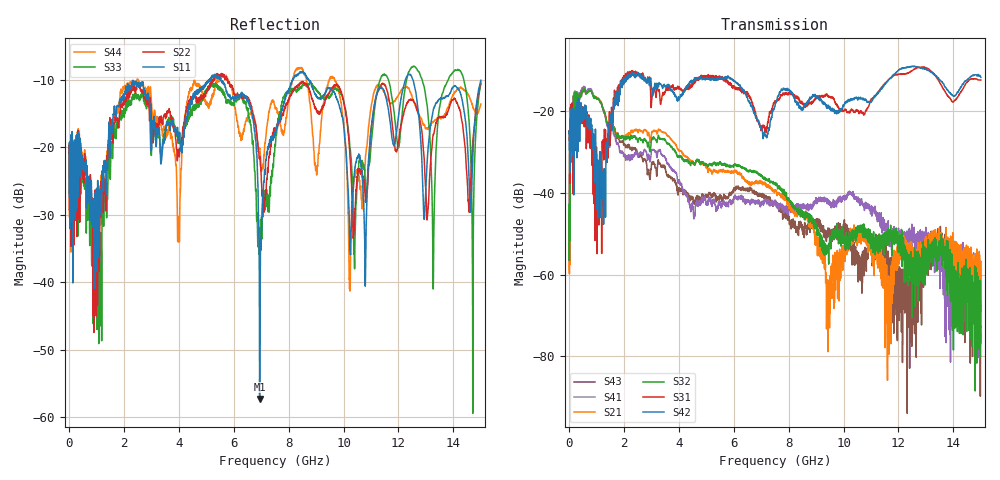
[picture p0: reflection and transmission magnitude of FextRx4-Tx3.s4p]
! FILE: N:\QM 2007\Prüfprotokolle\Highspeed\Konfektionierte Ltg\L45593-D106\D30\8216\0002\Fext\FextRx4-Tx3.s4p
# MHz S DB R 50.00
! FREQ  S11  S12  S13  S14
!  S21  S22  S23  S24
!  S31  S32  S33  S34
!  S41  S42  S43  S44
!  DB  ANG  DB  ANG  DB  ANG  DB  ANG
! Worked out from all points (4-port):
!   2999 points, 10 MHz to 15 GHz, reference 50 ohm
!   strongest paths, dB at 10 MHz, 3.755 GHz, 7.505 GHz, 11.26 GHz, 15 GHz:
!     S42: -25.4, -15.0, -18.7, -15.6, -11.6
!     S31: -24.8, -13.8, -17.8, -15.3, -12.3
!     S32: -42.9, -28.8, -37.8, -51.2, -76.7
!     S21: -46.8, -27.1, -39.3, -55.2, -67.4
!     S41: -58.8, -34.4, -42.0, -45.7, -68.1
!     S43: -45.1, -36.5, -42.2, -52.0, -65.3
!   lowest |S11| = -57.2 dB at 6.945 GHz (marker M1), VSWR 1.00, Z = 49.9 - j0.0939 ohm
!   |S11| at or under -10 dB: start of sweep to 5.119 GHz; 5.536 GHz to 8.151 GHz (2.615 GHz wide, 38.2 % of centre); 8.723 GHz to 12.25 GHz (3.529 GHz wide, 33.6 % of centre)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
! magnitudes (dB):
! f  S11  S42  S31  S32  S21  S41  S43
! 10 MHz  -19.4  -25.4  -24.8  -42.9  -46.8  -58.8  -45.1
! 535 MHz  -23.3  -21.4  -22.2  -14.6  -14.5  -14.1  -14.6
! 5.445 GHz  -9.7  -12.2  -11.5  -33.0  -34.5  -42.9  -41.3
! 6.945 GHz  -57.2  -23.5  -22.9  -35.4  -37.3  -42.0  -40.6
! 8.26 GHz  -9.5  -17.4  -16.3  -44.0  -45.4  -43.3  -48.7
! 10.22 GHz  -34.6  -17.5  -20.4  -51.4  -50.6  -39.7  -51.8
! 15 GHz  -10.1  -11.6  -12.3  -76.7  -67.4  -68.1  -65.3
